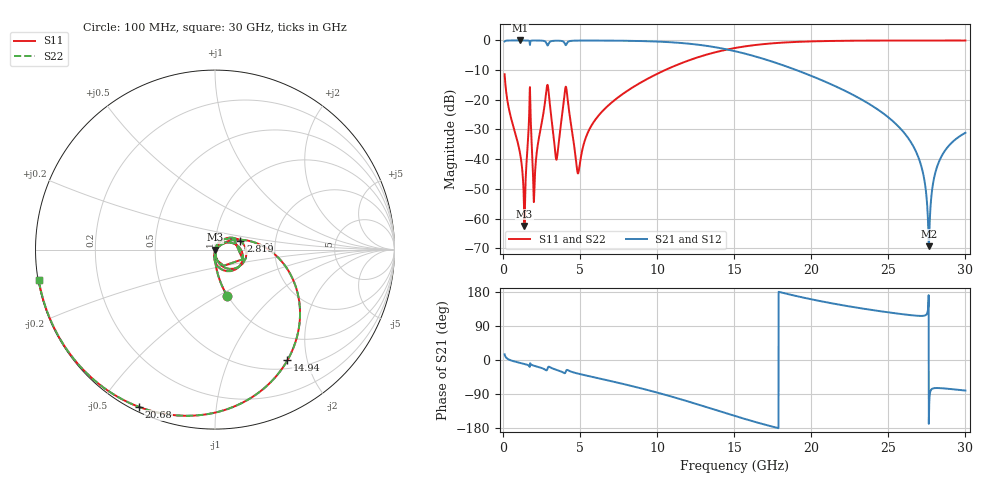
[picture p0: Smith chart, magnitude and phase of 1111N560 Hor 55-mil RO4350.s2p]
# GHz S MA R 50
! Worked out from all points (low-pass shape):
!   3201 points, 100 MHz to 30 GHz, reference 50 ohm
!   highest |S21| = -0.01 dB at 1.1 GHz (marker M1); lowest = -69.3 dB at 27.63 GHz (marker M2)
!   |S21| within 3 dB of the highest: start of sweep to 14.51 GHz
!   lowest |S11| = -62.5 dB at 1.389 GHz (marker M3), VSWR 1.00, Z = 50.1 - j0.00542 ohm
!   |S11| at or under -10 dB: start of sweep to 10.51 GHz
!   |S22| runs from -62.5 to 0.0 dB; largest |S21 - S12| = 0
!   S11 on the Smith chart (normalised r, x): 100 MHz: 0.99, -0.56; 2.819 GHz: 1.32, +0.13; 14.94 GHz: 0.62, -1.68; 20.68 GHz: 0.02, -0.63; 30 GHz: 0.00, -0.09
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0.1  0.2699 -75.1  0.9627 14.9  0.9627 14.9  0.2699 -75.1
1.099781  0.01263 -95.3  0.9993 -7.6  0.9993 -7.6  0.01263 -95.3
1.389438  0.0007514 -4.1  0.9991 -10.5  0.9991 -10.5  0.0007514 -4.1
1.688438  0.05085 60.0  0.9859 -15.5  0.9859 -15.5  0.05085 60.0
2.052844  0.00454 51.1  0.998 -15.7  0.998 -15.7  0.00454 51.1
2.819031  0.1495 19.1  0.8908 -27.3  0.8908 -27.3  0.1495 19.1
3.435719  0.01015 -36.7  0.9896 -25.5  0.9896 -25.5  0.01015 -36.7
4.071094  0.1662 -28.9  0.8334 -30.5  0.8334 -30.5  0.1662 -28.9
4.790563  0.006937 -61.1  0.9932 -35.2  0.9932 -35.2  0.006937 -61.1
5.089563  0.01229 30.0  0.9948 -38.1  0.9948 -38.1  0.01229 30.0
6.444406  0.06412 36.8  0.9942 -50.6  0.9942 -50.6  0.06412 36.8
10.06978  0.2795 2.6  0.9557 -86.7  0.9557 -86.7  0.2795 2.6
14.93788  0.7365 -56.7  0.6692 -146.4  0.6692 -146.4  0.7365 -56.7
15.05  0.7456 -58.1  0.659 -147.7  0.659 -147.7  0.7456 -58.1
20.03956  0.9644 -110.5  0.2506 159.9  0.2506 159.9  0.9644 -110.5
20.68428  0.9734 -115.8  0.2136 154.6  0.2136 154.6  0.9734 -115.8
25.01978  0.9958 -145.1  0.05017 125.6  0.05017 125.6  0.9958 -145.1
26.89787  0.997 -155.3  0.01162 116.7  0.01162 116.7  0.997 -155.3
27.29031  0.9971 -157.3  0.005199 116.7  0.005199 116.7  0.9971 -157.3
27.62669  0.9971 -159.0  0.0003419 -168.4  0.0003419 -168.4  0.9971 -159.0
28.31812  0.997 -162.4  0.009482 -74.1  0.009482 -74.1  0.997 -162.4
30  0.9966 -170.2  0.0278 -80.6  0.0278 -80.6  0.9966 -170.2
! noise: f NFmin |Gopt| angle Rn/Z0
0.1  0.0006248  0.72  1.633  0.0004418
3.417  0.02498  0.7589  25.51  0.01997
6.743  0.01938  0.4977  47.8  0.005683
10.06  0.02581  0.4755  65.52  0.00622
13.39  0.03743  0.5391  81.21  0.008842
16.7  0.05925  0.6576  98.04  0.01501
20.03  0.1089  0.7952  117.1  0.03097
23.35  0.26  0.9092  136.4  0.08805
26.67  1.614  0.9844  154.3  1.204
30  0.9273  0.9724  170.1  0.05816
